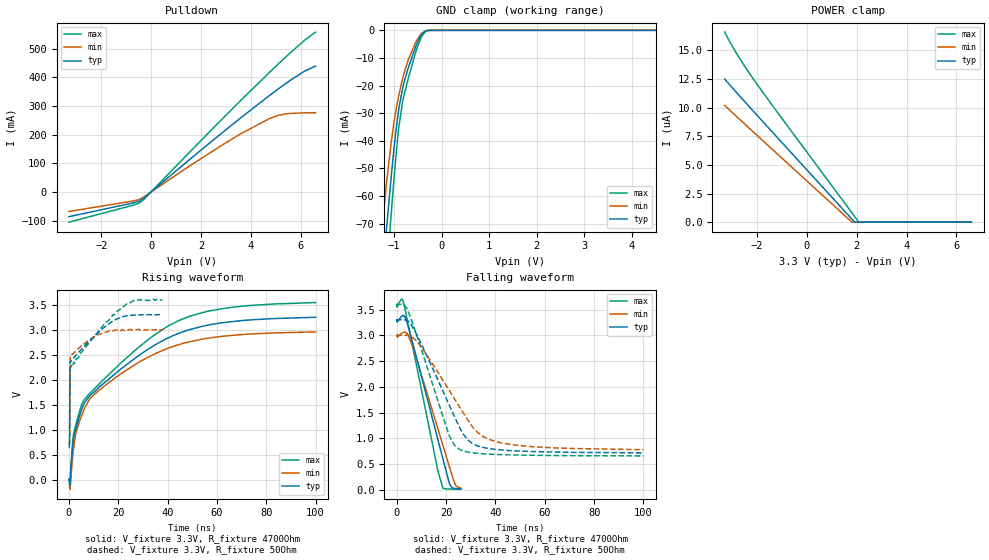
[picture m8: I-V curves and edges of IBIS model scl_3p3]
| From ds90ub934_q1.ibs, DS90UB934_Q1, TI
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|   scl_3p3 Model
[Model]   scl_3p3
Model_type   I/O_open_drain
Polarity   Non-Inverting
Vinl = 0.8
Vinh = 2.0
Vmeas = 1.65
Vref = 3.3
Cref = 550pF
Rref = 4700
|   typ   min   max
|   (nom PVT)   (fast PVT)   (slow PVT)
C_comp   1.660e-13   1.196e-13   2.265e-13
| Where nom  PVT is Nominal Process, 3.3V, 27C
|   Fast PVT is Strong Process,  3.6V, -40C
|   Slow PVT is Weak Process,   3V, 125C
[Voltage Range]   3.3   3   3.6
|Junction Temperature
[Temperature Range]   27   125   -40
[Pullup Reference]   3.3   3   3.6
[Pulldown Reference]   0   0   0
[Power Clamp Reference]   3.3   3   3.6
[GND Clamp Reference]   0   0   0
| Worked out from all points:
|   slope of the pulldown table from 0 to 0.495 V, typ, clamps not added: 13.6 ohm
|   GND clamp passes 1 mA (typ) near -0.39 V on its own axis
|   falling waveform, V_fixture 3.3V, R_fixture 4700Ohm: 20-80 % time 10.7ns typ, 11.3ns min, 9.11ns max; typ from 3.3 V to 0.015 V
|   rising waveform, V_fixture 3.3V, R_fixture 4700Ohm: 20-80 % time 30.3ns typ, 27.2ns min, 31.5ns max; typ from 0.01 V to 3.25 V
|   falling waveform, V_fixture 3.3V, R_fixture 50Ohm: 20-80 % time 14.8ns typ, 17.7ns min, 11.9ns max; typ from 3.3 V to 0.715 V
|   rising waveform, V_fixture 3.3V, R_fixture 50Ohm: 20-80 % time 8.05ns typ, 1.88ns min, 12.2ns max; typ from 0.706 V to 3.3 V
[Pulldown]
|   Voltage   I(typ)   I(min)   I(max)
-3.3V     -86.13mA   -68.1mA    -105.4mA
-702.9mV  -37.8mA    -31.02mA   -45.54mA
-481.8mV  -31.85mA   -26.05mA   -38.43mA
-330mV    -23.9mA    -19.31mA   -29.21mA
1.461V    107.1mA    85.88mA    131.6mA
2.832V    205.4mA    162.8mA    253mA
3.633V    261.4mA    205mA      322.7mA
4.743V    336.5mA    256.1mA    417.2mA
5.082V    358.5mA    267.2mA    445.3mA
5.388V    377.8mA    272.8mA    470.2mA
6.168V    422.5mA    276.4mA    530.4mA
6.6V      439.6mA    277mA      558.4mA
[GND Clamp]
|   Voltage   I(typ)   I(min)   I(max)
-3.3V     -551.9mA   -480.1mA   -622.9mA
-1.337V   -108.8mA   -86.72mA   -131.3mA
-1.226V   -86.04mA   -67.17mA   -105.1mA
-1.152V   -71.05mA   -54.74mA   -87.77mA
-1.068V   -54.85mA   -42.04mA   -68.68mA
-930.6mV  -32.38mA   -26.31mA   -40.4mA
-898.8mV  -28.5mA    -23.56mA   -35.11mA
-812.4mV  -20.47mA   -17.04mA   -25.22mA
-699mV    -13.54mA   -10.6mA    -17.36mA
-513.6mV  -4.647mA   -3.409mA   -6.339mA
-330mV    -193.3uA   -181.3uA   -287.3uA
6.6V      0A         0A         0A
[POWER Clamp]
|   Voltage   I(typ)   I(min)   I(max)
-3.3V     12.49uA    10.18uA    16.58uA
-3.044V   11.85uA    9.664uA    15.54uA
-2.756V   11.14uA    9.084uA    14.48uA
-2.025V   9.382uA    7.62uA     12.1uA
1.809V    255.2nA    0A         809.4nA
1.914V    0A         0A         501.4nA
2.082V    0A         0A         0A
6.6V      0A         0A         0A
[Ramp]
R_load = 4700
|   typ   min   max
dV/dt_r   1.9434/3.02838e-08   1.76747/2.71787e-08   2.12032/3.15469e-08
dV/dt_f   1.96144/1.0664e-08   1.7833/1.13233e-08   2.13784/9.04323e-09
[Falling Waveform]
V_fixture = 3.3V
V_fixture_min = 3V
V_fixture_max = 3.6V
R_fixture = 4700Ohm
|   Time   V(typ)   V(min)   V(max)
0s        3.3V       3V         3.6V
196.1ps   3.26V      2.983V     3.549V
2.039ns   3.373V     3.04V      3.705V
3.58ns    3.341V     3.057V     3.455V
6.378ns   2.863V     2.791V     2.799V
16.7ns    966.5mV    1.178V     358.3mV
18.7ns    597.5mV    860.6mV    25.37mV
21.56ns   90.71mV    410.8mV    12.01mV
23.9ns    22.08mV    85.1mV     10.5mV
25.95ns   15.23mV    30.63mV    9.969mV
[Rising Waveform]
V_fixture = 3.3V
V_fixture_min = 3V
V_fixture_max = 3.6V
R_fixture = 4700Ohm
|   Time   V(typ)   V(min)   V(max)
0s        9.536mV    10.71mV    8.512mV
358.9ps   -74.83mV   -36.46mV   -165mV
493.1ps   -60.41mV   -184.9mV   -22.49mV
1.831ns   789.1mV    603.9mV    891.8mV
2.878ns   1.031V     947.8mV    1.106V
6.125ns   1.518V     1.4V       1.598V
12.38ns   1.858V     1.797V     1.92V
32.7ns    2.629V     2.467V     2.824V
56.7ns    3.095V     2.833V     3.374V
100ns     3.249V     2.957V     3.542V
[Falling Waveform]
V_fixture = 3.3V
V_fixture_min = 3V
V_fixture_max = 3.6V
R_fixture = 50Ohm
|   Time   V(typ)   V(min)   V(max)
0s        3.3V       3V         3.6V
2.983ns   3.301V     3.001V     3.596V
6.175ns   3.181V     2.973V     3.266V
10.1ns    2.815V     2.762V     2.708V
21.42ns   1.628V     1.917V     1.037V
25.42ns   1.214V     1.61V      783.7mV
28.61ns   972.7mV    1.368V     733.9mV
32.49ns   857mV      1.124V     707.1mV
40.49ns   780.2mV    931mV      684.3mV
100ns     715.1mV    777.8mV    656mV
[Rising Waveform]
V_fixture = 3.3V
V_fixture_min = 3V
V_fixture_max = 3.6V
R_fixture = 50Ohm
|   Time   V(typ)   V(min)   V(max)
0s        705.9mV    757.9mV    653.5mV
230.5ps   710.1mV    745.8mV    695.2mV
309.1ps   819.5mV    782.6mV    1.548V
372.5ps   1.516V     897.6mV    2.144V
446.5ps   2.197V     1.579V     2.234V
534.6ps   2.366V     2.252V     2.254V
698.1ps   2.362V     2.477V     2.247V
12.1ns    2.955V     2.91V      2.976V
23.42ns   3.278V     2.994V     3.516V
37.92ns   3.298V     3V         3.586V
